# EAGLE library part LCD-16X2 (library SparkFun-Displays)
Standard text-only 16x2 parallel input LCD Basic 16 character by 2 line display. Typically utilizes the extremely common HD44780 parallel interface chipset SparkFun Products: Basic 16x2 Green Basic 8x2 Green
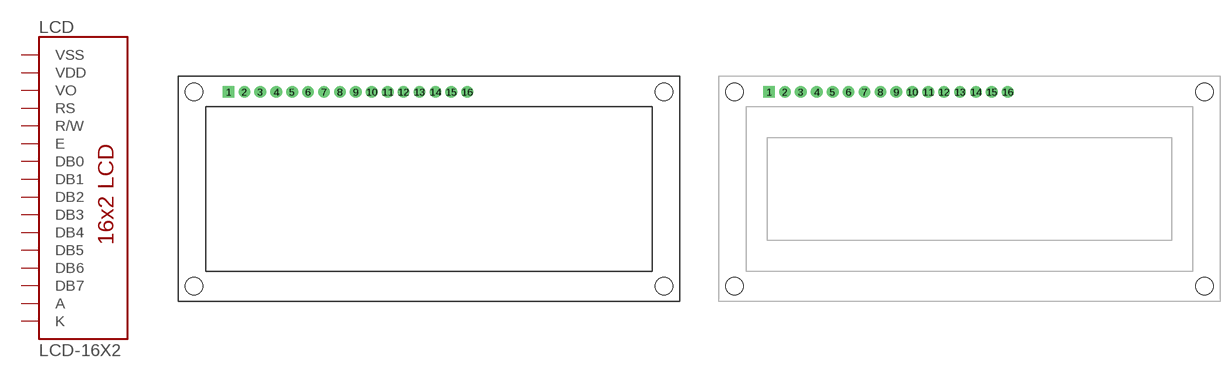
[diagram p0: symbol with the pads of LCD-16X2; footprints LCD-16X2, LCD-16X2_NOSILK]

Designator prefix LCD

## LCD-16X2SILK (PROD_ID: LCD-12633; SF_ID: LCD-00255)  [LCD-16X2]
1  VSS  pwr
2  VDD  pwr
3  VO
4  RS  in
5  R/W  in
6  E  in
7  DB0
8  DB1
9  DB2
10  DB3
11  DB4
12  DB5
13  DB6
14  DB7
15  A  pwr
16  K  pwr

## LCD-16X2NOSILK (SF_ID: LCD-00255)  [LCD-16X2_NOSILK]
Pads as for LCD-16X2

## LCD-16X2NOHOLES (SF_ID: LCD-00255)  [LCD-16X2_NOHOLESNOSILK]
Pads as for LCD-16X2

## LCD-16X28X2 (SF_ID: LCD-11122)  [LCD-8X2]
Pads as for LCD-16X2

## LCD-16X28X2-KIT (SF_ID: LCD-11122)  [LCD-8X2-KIT]
Pads as for LCD-16X2

## Footprint LCD-16X2 (pad centres in mm)
LCD-16x2 For Standard hitatchi type LCDs with backlight. Has 16 pin connection, silk outiline, and mounting holes. Specifications: Pin count: 16 Pin pitch: 0.1" Area: Datasheet referenced for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
drill 1.016 pad 1.88 square: 1 -32,15.5
drill 1.016 pad 1.88: 2 -29.46,15.5; 3 -26.92,15.5; 4 -24.38,15.5; 5 -21.84,15.5; 6 -19.3,15.5; 7 -16.76,15.5; 8 -14.22,15.5; 9 -11.68,15.5; 10 -9.14,15.5; 11 -6.6,15.5; 12 -4.06,15.5; 13 -1.52,15.5; 14 1.02,15.5; 15 3.56,15.5; 16 6.1,15.5
hole 2.8 at -37.5,15.5
hole 2.8 at -37.5,-15.5
hole 2.8 at 37.5,15.5
hole 2.8 at 37.5,-15.5

## Footprint LCD-16X2_NOSILK (pad centres in mm)
LCD-16x2 For Standard hitatchi type LCDs with backlight. Has 16 pin connection and outline on docu, and mounting holes, but no silkscreen. Specifications: Pin count: 16 Pin pitch: 0.1" Area: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
drill 1.016 pad 1.88 square: 1 -32,15.5
drill 1.016 pad 1.88: 2 -29.46,15.5; 3 -26.92,15.5; 4 -24.38,15.5; 5 -21.84,15.5; 6 -19.3,15.5; 7 -16.76,15.5; 8 -14.22,15.5; 9 -11.68,15.5; 10 -9.14,15.5; 11 -6.6,15.5; 12 -4.06,15.5; 13 -1.52,15.5; 14 1.02,15.5; 15 3.56,15.5; 16 6.1,15.5
hole 2.8 at -37.5,15.5
hole 2.8 at -37.5,-15.5
hole 2.8 at 37.5,15.5
hole 2.8 at 37.5,-15.5

## Footprint LCD-16X2_NOHOLESNOSILK (pad centres in mm)
LCD-16x2 No silk or mounting holes For Standard hitatchi type LCDs with backlight. Has 16 pin connection and outline on docu, but no silk or mounting holes. Specifications: Pin count: 16 Pin pitch: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
drill 1.016 pad 1.88 square: 1 -32,15.5
drill 1.016 pad 1.88: 2 -29.46,15.5; 3 -26.92,15.5; 4 -24.38,15.5; 5 -21.84,15.5; 6 -19.3,15.5; 7 -16.76,15.5; 8 -14.22,15.5; 9 -11.68,15.5; 10 -9.14,15.5; 11 -6.6,15.5; 12 -4.06,15.5; 13 -1.52,15.5; 14 1.02,15.5; 15 3.56,15.5; 16 6.1,15.5

## Footprint LCD-8X2 (pad centres in mm)
8x2 Character LCD w/ Backlight Specifications: Pin count: 16 Pin pitch: 0.1" Outer Dimensions: 40.0 x 35.4mm Viewing Area: 26.4 x 13.9mm Character Size: 2.95 x 4.75mm Datasheet referenced for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
drill 1 pad 1.778: 1 -7.62,13.73; 2 -7.62,16.27; 3 -5.08,13.73; 4 -5.08,16.27; 5 -2.54,13.73; 6 -2.54,16.27; 7 0,13.73; 8 0,16.27; 9 2.54,13.73; 10 2.54,16.27; 11 5.08,13.73; 12 5.08,16.27; 13 7.62,13.73; 14 7.62,16.27; 15 10.16,13.73; 16 10.16,16.27
hole 2 at 18,15
hole 2 at -18,15
hole 2 at -18,-15
hole 2 at 18,-15

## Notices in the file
Licensing: Creative Commons ShareAlike 4.0 International - https://creativecommons.org/licenses/by-sa/4.0
